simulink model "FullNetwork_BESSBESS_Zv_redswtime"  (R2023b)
settings: Solver=ode15s  StartTime=0.0  StopTime=140  RelTol=1e-3
PreLoadFcn:
  | Ts=50e-6;
model workspace (MAT data in the model file):
  Cf1 = 0.02
  Cf2 = 0.02
  Kffi1 = 0.9
  Kffi2 = 0.9
  Kffi3 = 0.9
  Kffv1 = 1
  Kffv2 = 1
  Kffv3 = 1
  Ki_cc1 = 5.9
  Ki_cc2 = 5.9
  Ki_cc3 = 5.9
  Ki_q1 = 0.0001
  Ki_q2 = 0.0001
  Ki_q3 = 0.0001
  Ki_vc1 = 150
  Ki_vc2 = 150
  Ki_vc3 = 150
  Kp_cc1 = 0.015
  Kp_cc2 = 0.015
  Kp_vc1 = 5
  Kp_vc2 = 5
  Kp_vc3 = 5
  Lf1 = 4.75e-06
  Lf2 = 4.75e-06
  Rf1 = 0.0005
  Rf2 = 0.0005
  Rf3 = 0.0005
  Rv1 = 0.0003169
  Rv2 = 0.0003169
  Snom1 = 100000000
  Snom2 = 100000000
  Vdc1 = 2000
  Vdc2 = 2000
  Vdc3 = 2000
  Xv1 = 0.0009509
  Xv2 = 0.0009509
  fnom1 = 50
  fnom2 = 50
  mp1 = 6.25e-08
  mp2 = 6.25e-08
  nq1 = 4.69166666667e-07
  nq2 = 4.69166666667e-07
  tau1 = 0.001
  tau2 = 0.001
  tau3 = 0.001
  vnom1 = 690
  vnom2 = 690
  vnom3 = 690
undefined symbols (not defined in the file or in its folder): Armidale, DiscIntNeverNeededParam, find_system, Gunnedah, Innerell, Ion, Lithium, Morree, Narrabri, Tamworth
libraries: spsThreePhaseBreakerLib x41, spsThreePhaseVIMeasurementLib x16, simulink_extras x16, spsThreePhaseSeriesRLCLoadLib x14, spsabctodq0Lib x12, spsThreePhaseTransformerTwoWindingsLib x11, slpidlib x8, spsLoadFlowBusLib x8, spsThreePhasePISectionLineLib x8, powerlib_extras x7, spsFirstOrderFilterLib x6, simulink x5
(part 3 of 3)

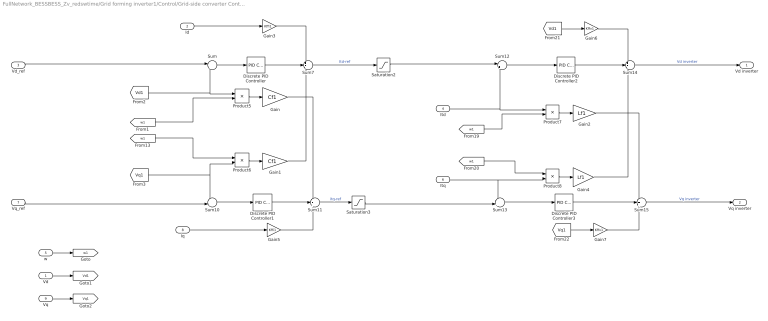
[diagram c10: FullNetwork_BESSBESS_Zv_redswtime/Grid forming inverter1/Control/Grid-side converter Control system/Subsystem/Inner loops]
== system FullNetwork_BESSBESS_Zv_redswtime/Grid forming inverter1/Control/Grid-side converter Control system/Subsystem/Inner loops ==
  Vd : Inport
  Id : Inport  Port=2
  Vd_ref : Inport  Port=3
  Itd : Inport  Port=4
  w : Inport  Port=5
  Itq : Inport  Port=6
  Vq_ref : Inport  Port=7
  Iq : Inport  Port=8
  Vq : Inport  Port=9
  Discrete PID Controller : slpidlib/PID Controller  Controller=PI  Form=Parallel  TimeDomain=Discrete-time  UseExternalTs=off  SampleTime=Ts  IntegratorMethod=Forward Euler  FilterMethod=Forward Euler  ControllerParametersSource=internal  P=Kp_vc1  I=Ki_vc1  UseKiTs=off  D=0  N=100  UseFilter=on  TunerSelectOption=Transfer Function Based (PID Tuner App)  InitialConditionSource=internal  InitialConditionForIntegrator=0  InitialConditionForFilter=0  DifferentiatorICPrevScaledInput=0  ExternalReset=none  TrackingMode=off  Kt=1  LimitOutput=off  SatLimitsSource=internal  UpperSaturationLimit=inf  LowerSaturationLimit=-inf  LinearizeAsGain=off  AntiWindupMode=none  Kb=1  LimitIntegrator=off  UpperIntegratorSaturationLimit=inf  LowerIntegratorSaturationLimit=-inf  POutMin=[]  POutMax=[]  IOutMin=[]  IOutMax=[]  DOutMin=[]  DOutMax=[]  NOutMin=[]  NOutMax=[]  SumOutMin=[]  SumOutMax=[]  SaturationOutMin=[]  SaturationOutMax=[]  PParamMin=[]  PParamMax=[]  IParamMin=[]  IParamMax=[]  DParamMin=[]  DParamMax=[]  NParamMin=[]  NParamMax=[]  KbParamMin=[]  KbParamMax=[]  KtParamMin=[]  KtParamMax=[]  KbOutMin=[]  KbOutMax=[]  KtOutMin=[]  KtOutMax=[]  IntegratorOutMin=[]  IntegratorOutMax=[]  FilterOutMin=[]  FilterOutMax=[]  SumI1OutMin=[]  SumI1OutMax=[]  SumI2OutMin=[]  SumI2OutMax=[]  SumI3OutMin=[]  SumI3OutMax=[]  SumI4OutMin=[]  SumI4OutMax=[]  SumDOutMin=[]  SumDOutMax=[]  DifferentiatorOutMin=[]  DifferentiatorOutMax=[]  FilterDiffOutCoefMin=[]  FilterDiffOutCoefMax=[]  ReciprocalOutMin=[]  ReciprocalOutMax=[]  SumDenOutMin=[]  SumDenOutMax=[]  SumNumOutMin=[]  SumNumOutMax=[]  DivideOutMin=[]  DivideOutMax=[]  UdiffTsProdOutMin=[]  UdiffTsProdOutMax=[]  NTsProdOutMin=[]  NTsProdOutMax=[]  UintegralTsProdOutMin=[]  UintegralTsProdOutMax=[]  UngainTsProdOutMin=[]  UngainTsProdOutMax=[]  ClampingZeroOutDataTypeStr=Inherit: Inherit via back propagation  ClampingZeroOutMin=[]  ClampingZeroOutMax=[]  FilterDenConstantOutDataTypeStr=Inherit: Inherit via back propagation  FilterDenConstantOutMin=[]  FilterDenConstantOutMax=[]  PCopyOutDataTypeStr=Inherit: Inherit via back propagation  PCopyOutMin=[]  PCopyOutMax=[]  NCopyOutDataTypeStr=Inherit: Inherit via back propagation  NCopyOutMin=[]  NCopyOutMax=[]  IntegratorContinuousStateAttributes=''  IntegratorStateMustResolveToSignalObject=off  IntegratorRTWStateStorageClass=Auto  FilterContinuousStateAttributes=''  FilterStateMustResolveToSignalObject=off  FilterRTWStateStorageClass=Auto  ParallelPVariant=InternalParameters  IdealPVariant=Disabled  IVariant=InternalParameters  DVariant=Disabled  IntegratorVariant=Discrete  SatVariant=Disabled  AWVariant=Passthrough  PCopyVariant=Disabled  TRVariant=Disabled  FdbkBlocksVariant=Forward  IdealPFdbkVariant=Disabled  SatFdbkVariant=Disabled  DerivativeFilterVariant=Disabled  NVariant=Disabled  NCopyVariant=Disabled_SignalSpec  FilterICVariant=Disabled  IntegratorICVariant=InternalICs  ExternalResetVariant=Disabled  TRSumVariant=Passthrough  SumFdbkVariant=Disabled  SumVariant=Sum_PI  TsampFilterVariant=InternalTs  TsampNgainVariant=Passthrough  TsampIntegralVariant=Disabled_SignalSpec  ExternalSaturationOutDataTypeStr=Inherit: Same as second input
  Discrete PID Controller1 : slpidlib/PID Controller  Controller=PI  Form=Parallel  TimeDomain=Discrete-time  UseExternalTs=off  SampleTime=Ts  IntegratorMethod=Forward Euler  FilterMethod=Forward Euler  ControllerParametersSource=internal  P=Kp_vc1  I=Ki_vc1  UseKiTs=off  D=0  N=100  UseFilter=on  TunerSelectOption=Transfer Function Based (PID Tuner App)  InitialConditionSource=internal  InitialConditionForIntegrator=0  InitialConditionForFilter=0  DifferentiatorICPrevScaledInput=0  ExternalReset=none  TrackingMode=off  Kt=1  LimitOutput=off  SatLimitsSource=internal  UpperSaturationLimit=inf  LowerSaturationLimit=-inf  LinearizeAsGain=off  AntiWindupMode=none  Kb=1  LimitIntegrator=off  UpperIntegratorSaturationLimit=inf  LowerIntegratorSaturationLimit=-inf  POutMin=[]  POutMax=[]  IOutMin=[]  IOutMax=[]  DOutMin=[]  DOutMax=[]  NOutMin=[]  NOutMax=[]  SumOutMin=[]  SumOutMax=[]  SaturationOutMin=[]  SaturationOutMax=[]  PParamMin=[]  PParamMax=[]  IParamMin=[]  IParamMax=[]  DParamMin=[]  DParamMax=[]  NParamMin=[]  NParamMax=[]  KbParamMin=[]  KbParamMax=[]  KtParamMin=[]  KtParamMax=[]  KbOutMin=[]  KbOutMax=[]  KtOutMin=[]  KtOutMax=[]  IntegratorOutMin=[]  IntegratorOutMax=[]  FilterOutMin=[]  FilterOutMax=[]  SumI1OutMin=[]  SumI1OutMax=[]  SumI2OutMin=[]  SumI2OutMax=[]  SumI3OutMin=[]  SumI3OutMax=[]  SumI4OutMin=[]  SumI4OutMax=[]  SumDOutMin=[]  SumDOutMax=[]  DifferentiatorOutMin=[]  DifferentiatorOutMax=[]  FilterDiffOutCoefMin=[]  FilterDiffOutCoefMax=[]  ReciprocalOutMin=[]  ReciprocalOutMax=[]  SumDenOutMin=[]  SumDenOutMax=[]  SumNumOutMin=[]  SumNumOutMax=[]  DivideOutMin=[]  DivideOutMax=[]  UdiffTsProdOutMin=[]  UdiffTsProdOutMax=[]  NTsProdOutMin=[]  NTsProdOutMax=[]  UintegralTsProdOutMin=[]  UintegralTsProdOutMax=[]  UngainTsProdOutMin=[]  UngainTsProdOutMax=[]  ClampingZeroOutDataTypeStr=Inherit: Inherit via back propagation  ClampingZeroOutMin=[]  ClampingZeroOutMax=[]  FilterDenConstantOutDataTypeStr=Inherit: Inherit via back propagation  FilterDenConstantOutMin=[]  FilterDenConstantOutMax=[]  PCopyOutDataTypeStr=Inherit: Inherit via back propagation  PCopyOutMin=[]  PCopyOutMax=[]  NCopyOutDataTypeStr=Inherit: Inherit via back propagation  NCopyOutMin=[]  NCopyOutMax=[]  IntegratorContinuousStateAttributes=''  IntegratorStateMustResolveToSignalObject=off  IntegratorRTWStateStorageClass=Auto  FilterContinuousStateAttributes=''  FilterStateMustResolveToSignalObject=off  FilterRTWStateStorageClass=Auto  ParallelPVariant=InternalParameters  IdealPVariant=Disabled  IVariant=InternalParameters  DVariant=Disabled  IntegratorVariant=Discrete  SatVariant=Disabled  AWVariant=Passthrough  PCopyVariant=Disabled  TRVariant=Disabled  FdbkBlocksVariant=Forward  IdealPFdbkVariant=Disabled  SatFdbkVariant=Disabled  DerivativeFilterVariant=Disabled  NVariant=Disabled  NCopyVariant=Disabled_SignalSpec  FilterICVariant=Disabled  IntegratorICVariant=InternalICs  ExternalResetVariant=Disabled  TRSumVariant=Passthrough  SumFdbkVariant=Disabled  SumVariant=Sum_PI  TsampFilterVariant=InternalTs  TsampNgainVariant=Passthrough  TsampIntegralVariant=Disabled_SignalSpec  ExternalSaturationOutDataTypeStr=Inherit: Same as second input
  Discrete PID Controller2 : slpidlib/PID Controller  Controller=PI  Form=Parallel  TimeDomain=Discrete-time  UseExternalTs=off  SampleTime=Ts  IntegratorMethod=Forward Euler  FilterMethod=Forward Euler  ControllerParametersSource=internal  P=Kp_cc1  I=Ki_cc1  UseKiTs=off  D=0  N=100  UseFilter=on  TunerSelectOption=Transfer Function Based (PID Tuner App)  InitialConditionSource=internal  InitialConditionForIntegrator=0  InitialConditionForFilter=0  DifferentiatorICPrevScaledInput=0  ExternalReset=none  TrackingMode=off  Kt=1  LimitOutput=off  SatLimitsSource=internal  UpperSaturationLimit=inf  LowerSaturationLimit=-inf  LinearizeAsGain=off  AntiWindupMode=none  Kb=1  LimitIntegrator=off  UpperIntegratorSaturationLimit=inf  LowerIntegratorSaturationLimit=-inf  POutMin=[]  POutMax=[]  IOutMin=[]  IOutMax=[]  DOutMin=[]  DOutMax=[]  NOutMin=[]  NOutMax=[]  SumOutMin=[]  SumOutMax=[]  SaturationOutMin=[]  SaturationOutMax=[]  PParamMin=[]  PParamMax=[]  IParamMin=[]  IParamMax=[]  DParamMin=[]  DParamMax=[]  NParamMin=[]  NParamMax=[]  KbParamMin=[]  KbParamMax=[]  KtParamMin=[]  KtParamMax=[]  KbOutMin=[]  KbOutMax=[]  KtOutMin=[]  KtOutMax=[]  IntegratorOutMin=[]  IntegratorOutMax=[]  FilterOutMin=[]  FilterOutMax=[]  SumI1OutMin=[]  SumI1OutMax=[]  SumI2OutMin=[]  SumI2OutMax=[]  SumI3OutMin=[]  SumI3OutMax=[]  SumI4OutMin=[]  SumI4OutMax=[]  SumDOutMin=[]  SumDOutMax=[]  DifferentiatorOutMin=[]  DifferentiatorOutMax=[]  FilterDiffOutCoefMin=[]  FilterDiffOutCoefMax=[]  ReciprocalOutMin=[]  ReciprocalOutMax=[]  SumDenOutMin=[]  SumDenOutMax=[]  SumNumOutMin=[]  SumNumOutMax=[]  DivideOutMin=[]  DivideOutMax=[]  UdiffTsProdOutMin=[]  UdiffTsProdOutMax=[]  NTsProdOutMin=[]  NTsProdOutMax=[]  UintegralTsProdOutMin=[]  UintegralTsProdOutMax=[]  UngainTsProdOutMin=[]  UngainTsProdOutMax=[]  ClampingZeroOutDataTypeStr=Inherit: Inherit via back propagation  ClampingZeroOutMin=[]  ClampingZeroOutMax=[]  FilterDenConstantOutDataTypeStr=Inherit: Inherit via back propagation  FilterDenConstantOutMin=[]  FilterDenConstantOutMax=[]  PCopyOutDataTypeStr=Inherit: Inherit via back propagation  PCopyOutMin=[]  PCopyOutMax=[]  NCopyOutDataTypeStr=Inherit: Inherit via back propagation  NCopyOutMin=[]  NCopyOutMax=[]  IntegratorContinuousStateAttributes=''  IntegratorStateMustResolveToSignalObject=off  IntegratorRTWStateStorageClass=Auto  FilterContinuousStateAttributes=''  FilterStateMustResolveToSignalObject=off  FilterRTWStateStorageClass=Auto  ParallelPVariant=InternalParameters  IdealPVariant=Disabled  IVariant=InternalParameters  DVariant=Disabled  IntegratorVariant=Discrete  SatVariant=Disabled  AWVariant=Passthrough  PCopyVariant=Disabled  TRVariant=Disabled  FdbkBlocksVariant=Forward  IdealPFdbkVariant=Disabled  SatFdbkVariant=Disabled  DerivativeFilterVariant=Disabled  NVariant=Disabled  NCopyVariant=Disabled_SignalSpec  FilterICVariant=Disabled  IntegratorICVariant=InternalICs  ExternalResetVariant=Disabled  TRSumVariant=Passthrough  SumFdbkVariant=Disabled  SumVariant=Sum_PI  TsampFilterVariant=InternalTs  TsampNgainVariant=Passthrough  TsampIntegralVariant=Disabled_SignalSpec  ExternalSaturationOutDataTypeStr=Inherit: Same as second input
  Discrete PID Controller3 : slpidlib/PID Controller  Controller=PI  Form=Parallel  TimeDomain=Discrete-time  UseExternalTs=off  SampleTime=Ts  IntegratorMethod=Forward Euler  FilterMethod=Forward Euler  ControllerParametersSource=internal  P=Kp_cc1  I=Ki_cc1  UseKiTs=off  D=0  N=100  UseFilter=on  TunerSelectOption=Transfer Function Based (PID Tuner App)  InitialConditionSource=internal  InitialConditionForIntegrator=0  InitialConditionForFilter=0  DifferentiatorICPrevScaledInput=0  ExternalReset=none  TrackingMode=off  Kt=1  LimitOutput=off  SatLimitsSource=internal  UpperSaturationLimit=inf  LowerSaturationLimit=-inf  LinearizeAsGain=off  AntiWindupMode=none  Kb=1  LimitIntegrator=off  UpperIntegratorSaturationLimit=inf  LowerIntegratorSaturationLimit=-inf  POutMin=[]  POutMax=[]  IOutMin=[]  IOutMax=[]  DOutMin=[]  DOutMax=[]  NOutMin=[]  NOutMax=[]  SumOutMin=[]  SumOutMax=[]  SaturationOutMin=[]  SaturationOutMax=[]  PParamMin=[]  PParamMax=[]  IParamMin=[]  IParamMax=[]  DParamMin=[]  DParamMax=[]  NParamMin=[]  NParamMax=[]  KbParamMin=[]  KbParamMax=[]  KtParamMin=[]  KtParamMax=[]  KbOutMin=[]  KbOutMax=[]  KtOutMin=[]  KtOutMax=[]  IntegratorOutMin=[]  IntegratorOutMax=[]  FilterOutMin=[]  FilterOutMax=[]  SumI1OutMin=[]  SumI1OutMax=[]  SumI2OutMin=[]  SumI2OutMax=[]  SumI3OutMin=[]  SumI3OutMax=[]  SumI4OutMin=[]  SumI4OutMax=[]  SumDOutMin=[]  SumDOutMax=[]  DifferentiatorOutMin=[]  DifferentiatorOutMax=[]  FilterDiffOutCoefMin=[]  FilterDiffOutCoefMax=[]  ReciprocalOutMin=[]  ReciprocalOutMax=[]  SumDenOutMin=[]  SumDenOutMax=[]  SumNumOutMin=[]  SumNumOutMax=[]  DivideOutMin=[]  DivideOutMax=[]  UdiffTsProdOutMin=[]  UdiffTsProdOutMax=[]  NTsProdOutMin=[]  NTsProdOutMax=[]  UintegralTsProdOutMin=[]  UintegralTsProdOutMax=[]  UngainTsProdOutMin=[]  UngainTsProdOutMax=[]  ClampingZeroOutDataTypeStr=Inherit: Inherit via back propagation  ClampingZeroOutMin=[]  ClampingZeroOutMax=[]  FilterDenConstantOutDataTypeStr=Inherit: Inherit via back propagation  FilterDenConstantOutMin=[]  FilterDenConstantOutMax=[]  PCopyOutDataTypeStr=Inherit: Inherit via back propagation  PCopyOutMin=[]  PCopyOutMax=[]  NCopyOutDataTypeStr=Inherit: Inherit via back propagation  NCopyOutMin=[]  NCopyOutMax=[]  IntegratorContinuousStateAttributes=''  IntegratorStateMustResolveToSignalObject=off  IntegratorRTWStateStorageClass=Auto  FilterContinuousStateAttributes=''  FilterStateMustResolveToSignalObject=off  FilterRTWStateStorageClass=Auto  ParallelPVariant=InternalParameters  IdealPVariant=Disabled  IVariant=InternalParameters  DVariant=Disabled  IntegratorVariant=Discrete  SatVariant=Disabled  AWVariant=Passthrough  PCopyVariant=Disabled  TRVariant=Disabled  FdbkBlocksVariant=Forward  IdealPFdbkVariant=Disabled  SatFdbkVariant=Disabled  DerivativeFilterVariant=Disabled  NVariant=Disabled  NCopyVariant=Disabled_SignalSpec  FilterICVariant=Disabled  IntegratorICVariant=InternalICs  ExternalResetVariant=Disabled  TRSumVariant=Passthrough  SumFdbkVariant=Disabled  SumVariant=Sum_PI  TsampFilterVariant=InternalTs  TsampNgainVariant=Passthrough  TsampIntegralVariant=Disabled_SignalSpec  ExternalSaturationOutDataTypeStr=Inherit: Same as second input
  Gain : Gain  Gain=Cf1
  Gain1 : Gain  Gain=Cf1
  Gain2 : Gain  Gain=Lf1
  Gain3 : Gain  Gain=Kffi1
  Gain4 : Gain  Gain=Lf1
  Gain5 : Gain  Gain=Kffi1
  Gain6 : Gain  Gain=Kffv1
  Gain7 : Gain  Gain=Kffv1
  Product{5..8} (4 alike) : Product
  Saturation2 : Saturate  UpperLimit=1.1*0.142*10e6  LowerLimit=-1.2*0.142*10e6  LinearizeAsGain=off  ZeroCross=off
  Saturation3 : Saturate  UpperLimit=1.1*0.106*10e6  LowerLimit=-1.2*0.106*10e6  LinearizeAsGain=off  ZeroCross=off
  Sum : Sum  Inputs=|+-
  Sum10 : Sum  Inputs=-+|
  Sum11 : Sum  Inputs=+++
  Sum12 : Sum  Inputs=|+-
  Sum13 : Sum  Inputs=-+|
  Sum14 : Sum  Inputs=++-
  Sum15 : Sum  Inputs=+++
  Sum7 : Sum  Inputs=++-
  Vd inverter : Outport
  Vq inverter : Outport  Port=2
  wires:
  [Vq1] -> Sum10/1, Product6/2
  Itd/1 -> Sum12/2, Product7/1
  Sum/1 -> Discrete PID Controller/1
  [w1] -> Product8/1
  Iq/1 -> Gain5/1
  Vd_ref/1 -> Sum/1
  [Vq1] -> Gain7/1
  Gain2/1 -> Sum15/1
  [Vd1] -> Gain6/1
  [Vd1] -> Sum/2, Product5/1
  Product5/1 -> Gain/1
  [w1] -> Product5/2
  Sum10/1 -> Discrete PID Controller1/1
  Gain3/1 -> Sum7/1
  Itq/1 -> Sum13/1, Product8/2
  Sum15/1 -> Vq inverter/1  "Vq inverter"
  [w1] -> Product6/1
  Product6/1 -> Gain1/1
  Gain/1 -> Sum11/1
  [w1] -> Product7/2
  Sum12/1 -> Discrete PID Controller2/1
  Vq_ref/1 -> Sum10/2
  Discrete PID Controller/1 -> Sum7/2
  Gain5/1 -> Sum11/3
  Gain4/1 -> Sum14/3
  Sum13/1 -> Discrete PID Controller3/1
  Gain1/1 -> Sum7/3
  Sum14/1 -> Vd inverter/1  "Vd inverter"
  Id/1 -> Gain3/1
  Product7/1 -> Gain2/1
  Product8/1 -> Gain4/1
  Discrete PID Controller2/1 -> Sum14/2
  Discrete PID Controller1/1 -> Sum11/2
  Gain6/1 -> Sum14/1
  Discrete PID Controller3/1 -> Sum15/2
  Gain7/1 -> Sum15/3
  w/1 -> [w1]
  Vd/1 -> [Vd1]
  Vq/1 -> [Vq1]
  Sum7/1 -> Saturation2/1  "Itd-ref"
  Saturation2/1 -> Sum12/1
  Sum11/1 -> Saturation3/1  "itq-ref"
  Saturation3/1 -> Sum13/2

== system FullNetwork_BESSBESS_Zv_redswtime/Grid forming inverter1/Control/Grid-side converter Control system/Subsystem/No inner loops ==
  Vd_ref : Inport
  Vq_ref : Inport  Port=2
  Vd inverter : Outport
  Vq inverter : Outport  Port=2
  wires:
  Vd_ref/1 -> Vd inverter/1
  Vq_ref/1 -> Vq inverter/1

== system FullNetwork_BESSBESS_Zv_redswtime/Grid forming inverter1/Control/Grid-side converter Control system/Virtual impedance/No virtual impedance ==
  Vd_ref : Inport
  Vq_ref : Inport  Port=2
  Vd_ref* : Outport
  Vq_ref* : Outport  Port=2
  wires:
  Vd_ref/1 -> Vd_ref*/1
  Vq_ref/1 -> Vq_ref*/1

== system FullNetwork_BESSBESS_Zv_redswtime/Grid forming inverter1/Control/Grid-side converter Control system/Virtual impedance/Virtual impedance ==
  Vd_ref : Inport
  Id : Inport  Port=2
  Iq : Inport  Port=3
  Vq_ref : Inport  Port=4
  Gain : Gain
  Gain1 : Gain
  Rvir1 : Gain  Gain=Xv1
  Rvir3 : Gain  Gain=Xv1
  Sum1 : Sum  Inputs=-+
  Sum11 : Sum  Inputs=|+-
  Sum12 : Sum  Inputs=-+
  Sum2 : Sum  Inputs=--
  Sum3 : Sum  Inputs=|++++
  Sum4 : Sum  Inputs=++++|
  T_power10 : powerlib_extras/Discrete  Control Blocks/Discrete 1st-Order Filter  FilterType=Lowpass  Tc=0.05  Ts=Ts  Initialize=on  Vac_Init=[0 0 0]  Vdc_Init=1  PlotResponse=off  param1=[1 200 0.1 ]
  T_power11 : powerlib_extras/Discrete  Control Blocks/Discrete 1st-Order Filter  FilterType=Lowpass  Tc=0.05  Ts=Ts  Initialize=on  Vac_Init=[0 0 0]  Vdc_Init=1  PlotResponse=off  param1=[1 200 0.1 ]
  T_power3 : powerlib_extras/Discrete  Control Blocks/Discrete 1st-Order Filter  FilterType=Lowpass  Tc=tau  Ts=Ts  Initialize=on  Vac_Init=[0 0 0]  Vdc_Init=1  PlotResponse=off  param1=[1 200 0.1]
  Transfer Fcn (with initial outputs){1..4} (4 alike) : simulink_extras/Additional Linear/Transfer Fcn (with initial outputs)  N=[0.2 0 ]  D=[0.2 1]  Y0=0  U0=0
  Xvir1 : Gain  Gain=Rv1
  Xvir2 : Gain  Gain=-10*Rv1
  Xvir3 : Gain  Gain=Rv1
  Xvir4 : Gain  Gain=-10*Rv1
  Xvir5 : Gain  Gain=10*Xv1
  Xvir6 : Gain  Gain=-10*Xv1
  Vd_ref* : Outport
  Vq_ref* : Outport  Port=2
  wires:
  Sum2/1 -> T_power11/1, Sum4/1
  Sum1/1 -> T_power10/1, Sum3/3
  Vq_ref/1 -> Sum4/2
  Vd_ref/1 -> Sum3/2
  Id/1 -> [Id1]
  Iq/1 -> [Iq1]
  [Id1] -> Xvir1/1
  Xvir1/1 -> Sum1/1
  [Iq1] -> Rvir3/1
  Rvir3/1 -> Sum1/2
  Rvir1/1 -> Sum2/1
  [Id1] -> Rvir1/1
  [Iq1] -> Xvir3/1
  Xvir3/1 -> Sum2/2
  Sum11/1 -> Vd_ref*/1
  Sum3/1 -> Sum11/1
  Sum12/1 -> Vq_ref*/1
  Sum4/1 -> Sum12/2
  T_power10/1 -> Gain/1
  Gain/1 -> Sum11/2
  T_power11/1 -> Gain1/1
  Gain1/1 -> Sum12/1
  Xvir2/1 -> Sum3/1
  Transfer Fcn (with initial outputs)1/1 -> Xvir2/1
  [Id1] -> Transfer Fcn (with initial outputs)1/1
  Xvir4/1 -> Sum4/3
  Transfer Fcn (with initial outputs)2/1 -> Xvir4/1
  [Iq1] -> Transfer Fcn (with initial outputs)2/1
  Transfer Fcn (with initial outputs)3/1 -> Xvir5/1
  [Iq1] -> Transfer Fcn (with initial outputs)3/1
  Xvir5/1 -> Sum3/4
  Transfer Fcn (with initial outputs)4/1 -> Xvir6/1
  [Id1] -> Transfer Fcn (with initial outputs)4/1
  Xvir6/1 -> Sum4/4

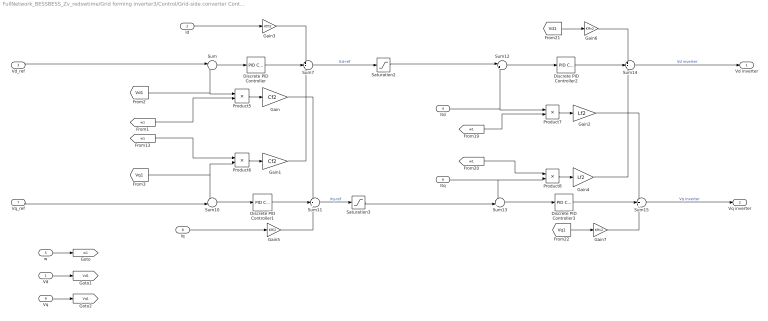
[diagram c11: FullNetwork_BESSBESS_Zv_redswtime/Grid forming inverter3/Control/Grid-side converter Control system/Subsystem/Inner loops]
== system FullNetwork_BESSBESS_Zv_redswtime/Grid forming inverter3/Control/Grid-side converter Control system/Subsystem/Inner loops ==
  Vd : Inport
  Id : Inport  Port=2
  Vd_ref : Inport  Port=3
  Itd : Inport  Port=4
  w : Inport  Port=5
  Itq : Inport  Port=6
  Vq_ref : Inport  Port=7
  Iq : Inport  Port=8
  Vq : Inport  Port=9
  Discrete PID Controller : slpidlib/PID Controller  Controller=PI  Form=Parallel  TimeDomain=Discrete-time  UseExternalTs=off  SampleTime=Ts  IntegratorMethod=Forward Euler  FilterMethod=Forward Euler  ControllerParametersSource=internal  P=Kp_vc2  I=Ki_vc2  UseKiTs=off  D=0  N=100  UseFilter=on  TunerSelectOption=Transfer Function Based (PID Tuner App)  InitialConditionSource=internal  InitialConditionForIntegrator=0  InitialConditionForFilter=0  DifferentiatorICPrevScaledInput=0  ExternalReset=none  TrackingMode=off  Kt=1  LimitOutput=off  SatLimitsSource=internal  UpperSaturationLimit=inf  LowerSaturationLimit=-inf  LinearizeAsGain=off  AntiWindupMode=none  Kb=1  LimitIntegrator=off  UpperIntegratorSaturationLimit=inf  LowerIntegratorSaturationLimit=-inf  POutMin=[]  POutMax=[]  IOutMin=[]  IOutMax=[]  DOutMin=[]  DOutMax=[]  NOutMin=[]  NOutMax=[]  SumOutMin=[]  SumOutMax=[]  SaturationOutMin=[]  SaturationOutMax=[]  PParamMin=[]  PParamMax=[]  IParamMin=[]  IParamMax=[]  DParamMin=[]  DParamMax=[]  NParamMin=[]  NParamMax=[]  KbParamMin=[]  KbParamMax=[]  KtParamMin=[]  KtParamMax=[]  KbOutMin=[]  KbOutMax=[]  KtOutMin=[]  KtOutMax=[]  IntegratorOutMin=[]  IntegratorOutMax=[]  FilterOutMin=[]  FilterOutMax=[]  SumI1OutMin=[]  SumI1OutMax=[]  SumI2OutMin=[]  SumI2OutMax=[]  SumI3OutMin=[]  SumI3OutMax=[]  SumI4OutMin=[]  SumI4OutMax=[]  SumDOutMin=[]  SumDOutMax=[]  DifferentiatorOutMin=[]  DifferentiatorOutMax=[]  FilterDiffOutCoefMin=[]  FilterDiffOutCoefMax=[]  ReciprocalOutMin=[]  ReciprocalOutMax=[]  SumDenOutMin=[]  SumDenOutMax=[]  SumNumOutMin=[]  SumNumOutMax=[]  DivideOutMin=[]  DivideOutMax=[]  UdiffTsProdOutMin=[]  UdiffTsProdOutMax=[]  NTsProdOutMin=[]  NTsProdOutMax=[]  UintegralTsProdOutMin=[]  UintegralTsProdOutMax=[]  UngainTsProdOutMin=[]  UngainTsProdOutMax=[]  ClampingZeroOutDataTypeStr=Inherit: Inherit via back propagation  ClampingZeroOutMin=[]  ClampingZeroOutMax=[]  FilterDenConstantOutDataTypeStr=Inherit: Inherit via back propagation  FilterDenConstantOutMin=[]  FilterDenConstantOutMax=[]  PCopyOutDataTypeStr=Inherit: Inherit via back propagation  PCopyOutMin=[]  PCopyOutMax=[]  NCopyOutDataTypeStr=Inherit: Inherit via back propagation  NCopyOutMin=[]  NCopyOutMax=[]  IntegratorContinuousStateAttributes=''  IntegratorStateMustResolveToSignalObject=off  IntegratorRTWStateStorageClass=Auto  FilterContinuousStateAttributes=''  FilterStateMustResolveToSignalObject=off  FilterRTWStateStorageClass=Auto  ParallelPVariant=InternalParameters  IdealPVariant=Disabled  IVariant=InternalParameters  DVariant=Disabled  IntegratorVariant=Discrete  SatVariant=Disabled  AWVariant=Passthrough  PCopyVariant=Disabled  TRVariant=Disabled  FdbkBlocksVariant=Forward  IdealPFdbkVariant=Disabled  SatFdbkVariant=Disabled  DerivativeFilterVariant=Disabled  NVariant=Disabled  NCopyVariant=Disabled_SignalSpec  FilterICVariant=Disabled  IntegratorICVariant=InternalICs  ExternalResetVariant=Disabled  TRSumVariant=Passthrough  SumFdbkVariant=Disabled  SumVariant=Sum_PI  TsampFilterVariant=InternalTs  TsampNgainVariant=Passthrough  TsampIntegralVariant=Disabled_SignalSpec  ExternalSaturationOutDataTypeStr=Inherit: Same as second input
  Discrete PID Controller1 : slpidlib/PID Controller  Controller=PI  Form=Parallel  TimeDomain=Discrete-time  UseExternalTs=off  SampleTime=Ts  IntegratorMethod=Forward Euler  FilterMethod=Forward Euler  ControllerParametersSource=internal  P=Kp_vc2  I=Ki_vc2  UseKiTs=off  D=0  N=100  UseFilter=on  TunerSelectOption=Transfer Function Based (PID Tuner App)  InitialConditionSource=internal  InitialConditionForIntegrator=0  InitialConditionForFilter=0  DifferentiatorICPrevScaledInput=0  ExternalReset=none  TrackingMode=off  Kt=1  LimitOutput=off  SatLimitsSource=internal  UpperSaturationLimit=inf  LowerSaturationLimit=-inf  LinearizeAsGain=off  AntiWindupMode=none  Kb=1  LimitIntegrator=off  UpperIntegratorSaturationLimit=inf  LowerIntegratorSaturationLimit=-inf  POutMin=[]  POutMax=[]  IOutMin=[]  IOutMax=[]  DOutMin=[]  DOutMax=[]  NOutMin=[]  NOutMax=[]  SumOutMin=[]  SumOutMax=[]  SaturationOutMin=[]  SaturationOutMax=[]  PParamMin=[]  PParamMax=[]  IParamMin=[]  IParamMax=[]  DParamMin=[]  DParamMax=[]  NParamMin=[]  NParamMax=[]  KbParamMin=[]  KbParamMax=[]  KtParamMin=[]  KtParamMax=[]  KbOutMin=[]  KbOutMax=[]  KtOutMin=[]  KtOutMax=[]  IntegratorOutMin=[]  IntegratorOutMax=[]  FilterOutMin=[]  FilterOutMax=[]  SumI1OutMin=[]  SumI1OutMax=[]  SumI2OutMin=[]  SumI2OutMax=[]  SumI3OutMin=[]  SumI3OutMax=[]  SumI4OutMin=[]  SumI4OutMax=[]  SumDOutMin=[]  SumDOutMax=[]  DifferentiatorOutMin=[]  DifferentiatorOutMax=[]  FilterDiffOutCoefMin=[]  FilterDiffOutCoefMax=[]  ReciprocalOutMin=[]  ReciprocalOutMax=[]  SumDenOutMin=[]  SumDenOutMax=[]  SumNumOutMin=[]  SumNumOutMax=[]  DivideOutMin=[]  DivideOutMax=[]  UdiffTsProdOutMin=[]  UdiffTsProdOutMax=[]  NTsProdOutMin=[]  NTsProdOutMax=[]  UintegralTsProdOutMin=[]  UintegralTsProdOutMax=[]  UngainTsProdOutMin=[]  UngainTsProdOutMax=[]  ClampingZeroOutDataTypeStr=Inherit: Inherit via back propagation  ClampingZeroOutMin=[]  ClampingZeroOutMax=[]  FilterDenConstantOutDataTypeStr=Inherit: Inherit via back propagation  FilterDenConstantOutMin=[]  FilterDenConstantOutMax=[]  PCopyOutDataTypeStr=Inherit: Inherit via back propagation  PCopyOutMin=[]  PCopyOutMax=[]  NCopyOutDataTypeStr=Inherit: Inherit via back propagation  NCopyOutMin=[]  NCopyOutMax=[]  IntegratorContinuousStateAttributes=''  IntegratorStateMustResolveToSignalObject=off  IntegratorRTWStateStorageClass=Auto  FilterContinuousStateAttributes=''  FilterStateMustResolveToSignalObject=off  FilterRTWStateStorageClass=Auto  ParallelPVariant=InternalParameters  IdealPVariant=Disabled  IVariant=InternalParameters  DVariant=Disabled  IntegratorVariant=Discrete  SatVariant=Disabled  AWVariant=Passthrough  PCopyVariant=Disabled  TRVariant=Disabled  FdbkBlocksVariant=Forward  IdealPFdbkVariant=Disabled  SatFdbkVariant=Disabled  DerivativeFilterVariant=Disabled  NVariant=Disabled  NCopyVariant=Disabled_SignalSpec  FilterICVariant=Disabled  IntegratorICVariant=InternalICs  ExternalResetVariant=Disabled  TRSumVariant=Passthrough  SumFdbkVariant=Disabled  SumVariant=Sum_PI  TsampFilterVariant=InternalTs  TsampNgainVariant=Passthrough  TsampIntegralVariant=Disabled_SignalSpec  ExternalSaturationOutDataTypeStr=Inherit: Same as second input
  Discrete PID Controller2 : slpidlib/PID Controller  Controller=PI  Form=Parallel  TimeDomain=Discrete-time  UseExternalTs=off  SampleTime=Ts  IntegratorMethod=Forward Euler  FilterMethod=Forward Euler  ControllerParametersSource=internal  P=Kp_cc2  I=Ki_cc2  UseKiTs=off  D=0  N=100  UseFilter=on  TunerSelectOption=Transfer Function Based (PID Tuner App)  InitialConditionSource=internal  InitialConditionForIntegrator=0  InitialConditionForFilter=0  DifferentiatorICPrevScaledInput=0  ExternalReset=none  TrackingMode=off  Kt=1  LimitOutput=off  SatLimitsSource=internal  UpperSaturationLimit=inf  LowerSaturationLimit=-inf  LinearizeAsGain=off  AntiWindupMode=none  Kb=1  LimitIntegrator=off  UpperIntegratorSaturationLimit=inf  LowerIntegratorSaturationLimit=-inf  POutMin=[]  POutMax=[]  IOutMin=[]  IOutMax=[]  DOutMin=[]  DOutMax=[]  NOutMin=[]  NOutMax=[]  SumOutMin=[]  SumOutMax=[]  SaturationOutMin=[]  SaturationOutMax=[]  PParamMin=[]  PParamMax=[]  IParamMin=[]  IParamMax=[]  DParamMin=[]  DParamMax=[]  NParamMin=[]  NParamMax=[]  KbParamMin=[]  KbParamMax=[]  KtParamMin=[]  KtParamMax=[]  KbOutMin=[]  KbOutMax=[]  KtOutMin=[]  KtOutMax=[]  IntegratorOutMin=[]  IntegratorOutMax=[]  FilterOutMin=[]  FilterOutMax=[]  SumI1OutMin=[]  SumI1OutMax=[]  SumI2OutMin=[]  SumI2OutMax=[]  SumI3OutMin=[]  SumI3OutMax=[]  SumI4OutMin=[]  SumI4OutMax=[]  SumDOutMin=[]  SumDOutMax=[]  DifferentiatorOutMin=[]  DifferentiatorOutMax=[]  FilterDiffOutCoefMin=[]  FilterDiffOutCoefMax=[]  ReciprocalOutMin=[]  ReciprocalOutMax=[]  SumDenOutMin=[]  SumDenOutMax=[]  SumNumOutMin=[]  SumNumOutMax=[]  DivideOutMin=[]  DivideOutMax=[]  UdiffTsProdOutMin=[]  UdiffTsProdOutMax=[]  NTsProdOutMin=[]  NTsProdOutMax=[]  UintegralTsProdOutMin=[]  UintegralTsProdOutMax=[]  UngainTsProdOutMin=[]  UngainTsProdOutMax=[]  ClampingZeroOutDataTypeStr=Inherit: Inherit via back propagation  ClampingZeroOutMin=[]  ClampingZeroOutMax=[]  FilterDenConstantOutDataTypeStr=Inherit: Inherit via back propagation  FilterDenConstantOutMin=[]  FilterDenConstantOutMax=[]  PCopyOutDataTypeStr=Inherit: Inherit via back propagation  PCopyOutMin=[]  PCopyOutMax=[]  NCopyOutDataTypeStr=Inherit: Inherit via back propagation  NCopyOutMin=[]  NCopyOutMax=[]  IntegratorContinuousStateAttributes=''  IntegratorStateMustResolveToSignalObject=off  IntegratorRTWStateStorageClass=Auto  FilterContinuousStateAttributes=''  FilterStateMustResolveToSignalObject=off  FilterRTWStateStorageClass=Auto  ParallelPVariant=InternalParameters  IdealPVariant=Disabled  IVariant=InternalParameters  DVariant=Disabled  IntegratorVariant=Discrete  SatVariant=Disabled  AWVariant=Passthrough  PCopyVariant=Disabled  TRVariant=Disabled  FdbkBlocksVariant=Forward  IdealPFdbkVariant=Disabled  SatFdbkVariant=Disabled  DerivativeFilterVariant=Disabled  NVariant=Disabled  NCopyVariant=Disabled_SignalSpec  FilterICVariant=Disabled  IntegratorICVariant=InternalICs  ExternalResetVariant=Disabled  TRSumVariant=Passthrough  SumFdbkVariant=Disabled  SumVariant=Sum_PI  TsampFilterVariant=InternalTs  TsampNgainVariant=Passthrough  TsampIntegralVariant=Disabled_SignalSpec  ExternalSaturationOutDataTypeStr=Inherit: Same as second input
  Discrete PID Controller3 : slpidlib/PID Controller  Controller=PI  Form=Parallel  TimeDomain=Discrete-time  UseExternalTs=off  SampleTime=Ts  IntegratorMethod=Forward Euler  FilterMethod=Forward Euler  ControllerParametersSource=internal  P=Kp_cc2  I=Ki_cc2  UseKiTs=off  D=0  N=100  UseFilter=on  TunerSelectOption=Transfer Function Based (PID Tuner App)  InitialConditionSource=internal  InitialConditionForIntegrator=0  InitialConditionForFilter=0  DifferentiatorICPrevScaledInput=0  ExternalReset=none  TrackingMode=off  Kt=1  LimitOutput=off  SatLimitsSource=internal  UpperSaturationLimit=inf  LowerSaturationLimit=-inf  LinearizeAsGain=off  AntiWindupMode=none  Kb=1  LimitIntegrator=off  UpperIntegratorSaturationLimit=inf  LowerIntegratorSaturationLimit=-inf  POutMin=[]  POutMax=[]  IOutMin=[]  IOutMax=[]  DOutMin=[]  DOutMax=[]  NOutMin=[]  NOutMax=[]  SumOutMin=[]  SumOutMax=[]  SaturationOutMin=[]  SaturationOutMax=[]  PParamMin=[]  PParamMax=[]  IParamMin=[]  IParamMax=[]  DParamMin=[]  DParamMax=[]  NParamMin=[]  NParamMax=[]  KbParamMin=[]  KbParamMax=[]  KtParamMin=[]  KtParamMax=[]  KbOutMin=[]  KbOutMax=[]  KtOutMin=[]  KtOutMax=[]  IntegratorOutMin=[]  IntegratorOutMax=[]  FilterOutMin=[]  FilterOutMax=[]  SumI1OutMin=[]  SumI1OutMax=[]  SumI2OutMin=[]  SumI2OutMax=[]  SumI3OutMin=[]  SumI3OutMax=[]  SumI4OutMin=[]  SumI4OutMax=[]  SumDOutMin=[]  SumDOutMax=[]  DifferentiatorOutMin=[]  DifferentiatorOutMax=[]  FilterDiffOutCoefMin=[]  FilterDiffOutCoefMax=[]  ReciprocalOutMin=[]  ReciprocalOutMax=[]  SumDenOutMin=[]  SumDenOutMax=[]  SumNumOutMin=[]  SumNumOutMax=[]  DivideOutMin=[]  DivideOutMax=[]  UdiffTsProdOutMin=[]  UdiffTsProdOutMax=[]  NTsProdOutMin=[]  NTsProdOutMax=[]  UintegralTsProdOutMin=[]  UintegralTsProdOutMax=[]  UngainTsProdOutMin=[]  UngainTsProdOutMax=[]  ClampingZeroOutDataTypeStr=Inherit: Inherit via back propagation  ClampingZeroOutMin=[]  ClampingZeroOutMax=[]  FilterDenConstantOutDataTypeStr=Inherit: Inherit via back propagation  FilterDenConstantOutMin=[]  FilterDenConstantOutMax=[]  PCopyOutDataTypeStr=Inherit: Inherit via back propagation  PCopyOutMin=[]  PCopyOutMax=[]  NCopyOutDataTypeStr=Inherit: Inherit via back propagation  NCopyOutMin=[]  NCopyOutMax=[]  IntegratorContinuousStateAttributes=''  IntegratorStateMustResolveToSignalObject=off  IntegratorRTWStateStorageClass=Auto  FilterContinuousStateAttributes=''  FilterStateMustResolveToSignalObject=off  FilterRTWStateStorageClass=Auto  ParallelPVariant=InternalParameters  IdealPVariant=Disabled  IVariant=InternalParameters  DVariant=Disabled  IntegratorVariant=Discrete  SatVariant=Disabled  AWVariant=Passthrough  PCopyVariant=Disabled  TRVariant=Disabled  FdbkBlocksVariant=Forward  IdealPFdbkVariant=Disabled  SatFdbkVariant=Disabled  DerivativeFilterVariant=Disabled  NVariant=Disabled  NCopyVariant=Disabled_SignalSpec  FilterICVariant=Disabled  IntegratorICVariant=InternalICs  ExternalResetVariant=Disabled  TRSumVariant=Passthrough  SumFdbkVariant=Disabled  SumVariant=Sum_PI  TsampFilterVariant=InternalTs  TsampNgainVariant=Passthrough  TsampIntegralVariant=Disabled_SignalSpec  ExternalSaturationOutDataTypeStr=Inherit: Same as second input
  Gain : Gain  Gain=Cf2
  Gain1 : Gain  Gain=Cf2
  Gain2 : Gain  Gain=Lf2
  Gain3 : Gain  Gain=Kffi2
  Gain4 : Gain  Gain=Lf2
  Gain5 : Gain  Gain=Kffi2
  Gain6 : Gain  Gain=Kffv2
  Gain7 : Gain  Gain=Kffv2
  Product{5..8} (4 alike) : Product
  Saturation2 : Saturate  UpperLimit=1.2*0.142*10e6  LowerLimit=-1.2*0.142*10e6  LinearizeAsGain=off  ZeroCross=off
  Saturation3 : Saturate  UpperLimit=1.2*0.106*10e6  LowerLimit=-1.2*0.106*10e6  LinearizeAsGain=off  ZeroCross=off
  Sum : Sum  Inputs=|+-
  Sum10 : Sum  Inputs=-+|
  Sum11 : Sum  Inputs=+++
  Sum12 : Sum  Inputs=|+-
  Sum13 : Sum  Inputs=-+|
  Sum14 : Sum  Inputs=++-
  Sum15 : Sum  Inputs=+++
  Sum7 : Sum  Inputs=++-
  Vd inverter : Outport
  Vq inverter : Outport  Port=2
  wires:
  [Vq1] -> Sum10/1, Product6/2
  Itd/1 -> Sum12/2, Product7/1
  Sum/1 -> Discrete PID Controller/1
  [w1] -> Product8/1
  Iq/1 -> Gain5/1
  Vd_ref/1 -> Sum/1
  [Vq1] -> Gain7/1
  Gain2/1 -> Sum15/1
  [Vd1] -> Gain6/1
  [Vd1] -> Sum/2, Product5/1
  Product5/1 -> Gain/1
  [w1] -> Product5/2
  Sum10/1 -> Discrete PID Controller1/1
  Gain3/1 -> Sum7/1
  Itq/1 -> Sum13/1, Product8/2
  Sum15/1 -> Vq inverter/1  "Vq inverter"
  [w1] -> Product6/1
  Product6/1 -> Gain1/1
  Gain/1 -> Sum11/1
  [w1] -> Product7/2
  Sum12/1 -> Discrete PID Controller2/1
  Vq_ref/1 -> Sum10/2
  Discrete PID Controller/1 -> Sum7/2
  Gain5/1 -> Sum11/3
  Gain4/1 -> Sum14/3
  Sum13/1 -> Discrete PID Controller3/1
  Gain1/1 -> Sum7/3
  Sum14/1 -> Vd inverter/1  "Vd inverter"
  Id/1 -> Gain3/1
  Product7/1 -> Gain2/1
  Product8/1 -> Gain4/1
  Discrete PID Controller2/1 -> Sum14/2
  Discrete PID Controller1/1 -> Sum11/2
  Gain6/1 -> Sum14/1
  Discrete PID Controller3/1 -> Sum15/2
  Gain7/1 -> Sum15/3
  w/1 -> [w1]
  Vd/1 -> [Vd1]
  Vq/1 -> [Vq1]
  Sum7/1 -> Saturation2/1  "Itd-ref"
  Saturation2/1 -> Sum12/1
  Sum11/1 -> Saturation3/1  "itq-ref"
  Saturation3/1 -> Sum13/2

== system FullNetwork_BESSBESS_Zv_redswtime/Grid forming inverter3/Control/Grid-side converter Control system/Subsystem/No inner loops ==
  Vd_ref : Inport
  Vq_ref : Inport  Port=2
  Vd inverter : Outport
  Vq inverter : Outport  Port=2
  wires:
  Vd_ref/1 -> Vd inverter/1
  Vq_ref/1 -> Vq inverter/1

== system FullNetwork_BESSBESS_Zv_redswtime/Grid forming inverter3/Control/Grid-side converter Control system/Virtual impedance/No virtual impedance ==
  Vd_ref : Inport
  Vq_ref : Inport  Port=2
  Vd_ref* : Outport
  Vq_ref* : Outport  Port=2
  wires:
  Vd_ref/1 -> Vd_ref*/1
  Vq_ref/1 -> Vq_ref*/1

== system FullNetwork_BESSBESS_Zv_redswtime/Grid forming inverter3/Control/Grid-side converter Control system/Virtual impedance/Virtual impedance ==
  Vd_ref : Inport
  Id : Inport  Port=2
  Iq : Inport  Port=3
  Vq_ref : Inport  Port=4
  Rvir1 : Gain  Gain=Xv2
  Rvir2 : Gain  Gain=10*Xv2
  Rvir3 : Gain  Gain=Xv2
  Rvir4 : Gain  Gain=10*Xv2
  Sum1 : Sum  Inputs=-+
  Sum2 : Sum  Inputs=--
  Sum3 : Sum  Inputs=|++++
  Sum4 : Sum  Inputs=+++|
  Sum5 : Sum  Inputs=|+-
  Sum6 : Sum  Inputs=|-+
  Sum7 : Sum  Inputs=-+
  Sum8 : Sum  Inputs=--
  T_power10 : powerlib_extras/Discrete  Control Blocks/Discrete 1st-Order Filter  FilterType=Lowpass  Tc=0.05  Ts=Ts  Initialize=on  Vac_Init=[0 0 0]  Vdc_Init=1  PlotResponse=off  param1=[1 200 0.1 ]
  T_power4 : powerlib_extras/Discrete  Control Blocks/Discrete 1st-Order Filter  FilterType=Lowpass  Tc=0.05  Ts=Ts  Initialize=on  Vac_Init=[0 0 0]  Vdc_Init=1  PlotResponse=off  param1=[1 200 0.1 ]
  Transfer Fcn (with initial outputs){1..4} (4 alike) : simulink_extras/Additional Linear/Transfer Fcn (with initial outputs)  N=[0.5*0.2 0 ]  D=[0.2 1]  Y0=0  U0=0
  Xvir1 : Gain  Gain=Rv2
  Xvir2 : Gain  Gain=10*Rv2
  Xvir3 : Gain  Gain=Rv2
  Xvir4 : Gain  Gain=10*Rv2
  Vd_ref* : Outport
  Vq_ref* : Outport  Port=2
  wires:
  Sum1/1 -> Sum3/4, T_power10/1
  Vq_ref/1 -> Sum4/2
  Id/1 -> [Id2]
  Iq/1 -> [Iq2]
  [Id2] -> Xvir1/1
  Xvir1/1 -> Sum1/1
  [Iq2] -> Rvir3/1
  Rvir3/1 -> Sum1/2
  Rvir1/1 -> Sum2/1
  [Id2] -> Rvir1/1
  [Iq2] -> Xvir3/1
  Xvir3/1 -> Sum2/2
  Sum5/1 -> Vd_ref*/1
  Sum3/1 -> Sum5/1
  Sum2/1 -> T_power4/1, Sum4/1
  Sum4/1 -> Sum6/2
  Sum6/1 -> Vq_ref*/1
  Vd_ref/1 -> Sum3/2
  Rvir2/1 -> Sum7/2
  Xvir2/1 -> Sum7/1
  Xvir4/1 -> Sum8/2
  Rvir4/1 -> Sum8/1
  Transfer Fcn (with initial outputs)2/1 -> Xvir2/1
  [Id2] -> Transfer Fcn (with initial outputs)2/1
  [Iq2] -> Transfer Fcn (with initial outputs)1/1
  Transfer Fcn (with initial outputs)1/1 -> Rvir2/1
  [Id2] -> Transfer Fcn (with initial outputs)3/1
  Transfer Fcn (with initial outputs)3/1 -> Rvir4/1
  [Iq2] -> Transfer Fcn (with initial outputs)4/1
  Transfer Fcn (with initial outputs)4/1 -> Xvir4/1
  T_power10/1 -> Sum5/2
  T_power4/1 -> Sum6/1
  Sum8/1 -> Sum4/3
  Sum7/1 -> Sum3/1
